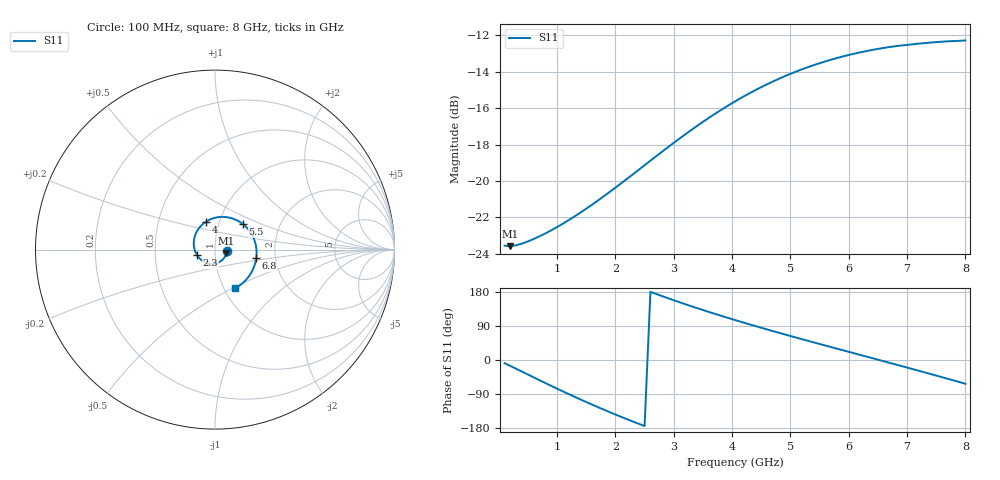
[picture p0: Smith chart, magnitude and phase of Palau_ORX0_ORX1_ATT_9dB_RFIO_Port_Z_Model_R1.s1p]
! Created Fri Oct  9 14:29:32 2020
! Palau ORX0/ORX1 RFIO Port Impedance Model.
! Attenuation  : 9 dB.
! Revision		: R1.
! Impedance Mode 	: Balanced Differential-Mode.
! Impedance Format 	: Series Equivalent Differential Impedance (SEDZ).
# hz S ma R 100
! 1 Port Network Data from SP1.SP block
! freq  magS11  angS11
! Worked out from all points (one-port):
!   80 points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, 100 MHz to 8 GHz, reference 100 ohm
!   lowest |S11| = -23.6 dB at 200 MHz (marker M1), VSWR 1.14, Z = 114 - j4.12 ohm
!   |S11| at or under -10 dB: start of sweep to end of sweep
!   S11 on the Smith chart (normalised r, x): 100 MHz: 1.14, -0.02; 2.3 GHz: 0.82, -0.05; 4 GHz: 0.86, +0.28; 5.5 GHz: 1.30, +0.39; 6.8 GHz: 1.59, -0.16; 8 GHz: 1.12, -0.52
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1e8  0.06632 -8.5
2e8  0.06613 -15.9
6e8  0.06922 -45.9
1.1e9  0.07628 -82.9
1.4e9  0.08181 -104.1
1.6e9  0.08603 -117.7
1.8e9  0.0907 -131.0
2.1e9  0.09853 -150.1
2.3e9  0.1043 -162.4
2.7e9  0.117 174.3
3.1e9  0.1308 152.4
3.5e9  0.1453 131.9
3.7e9  0.1527 122.0
4e9  0.1636 107.8
4.1e9  0.1672 103.2
4.4e9  0.1777 89.5
4.6e9  0.1844 80.7
4.9e9  0.194 67.7
5.1e9  0.1999 59.1
5.5e9  0.2107 42.3
5.8e9  0.2178 29.8
6.1e9  0.224 17.4
6.5e9  0.2307 0.9
6.8e9  0.2347 -11.6
7.1e9  0.2376 -24.1
7.5e9  0.2409 -41.1
7.7e9  0.2421 -49.7
8e9  0.2434 -62.8
